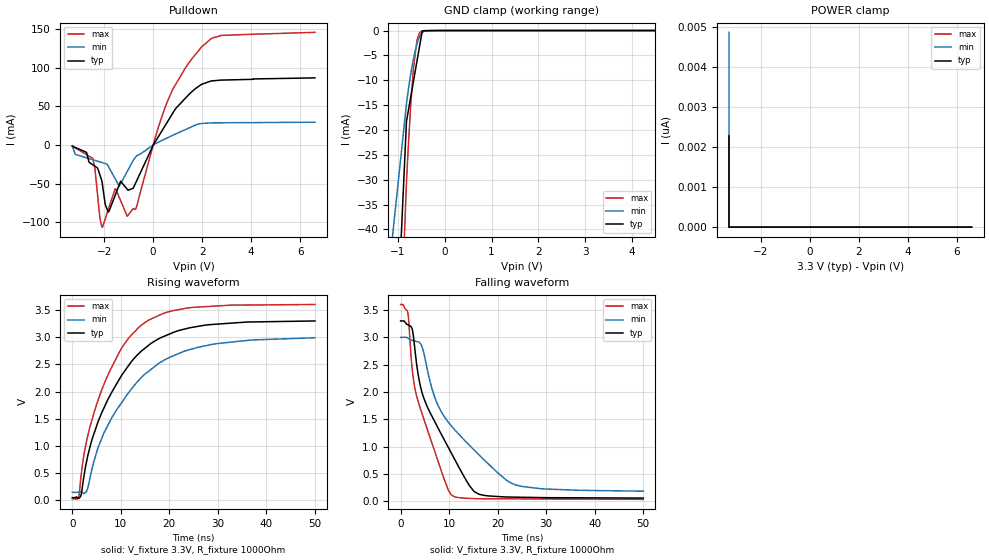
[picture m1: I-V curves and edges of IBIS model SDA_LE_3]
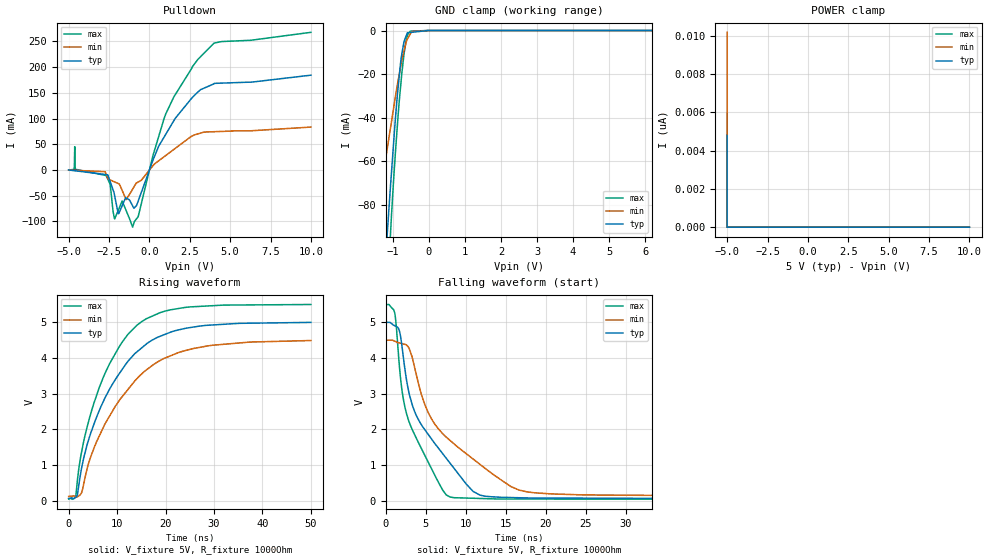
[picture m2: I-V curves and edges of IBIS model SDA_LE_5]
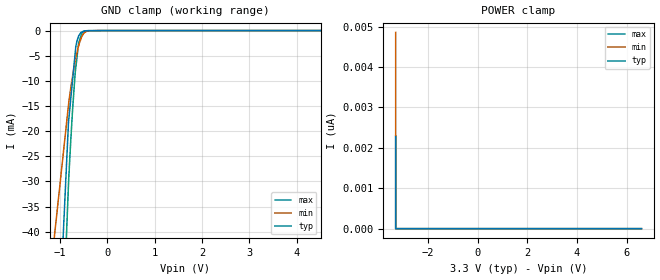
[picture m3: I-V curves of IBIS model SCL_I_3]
| Texas Instruments Incorporated
| Low-Power Bidirectional I2C Isolators
| Marketing part#   Voltage Range   Package-type   #pins/pkg drawing
| ISO1541D   3V-5.5V   SOIC   8-pin D
[IBIS Ver]   4.1
[File name]   iso1541.ibs
[File Rev]   1.0
[Date]   06/21/2012
[Source]   TIspiceD simulations
   Texas Instruments Incorporated.
   Analog eLab Design Center, HPA
   12500 TI Blvd
   Dallas, TX -75243
   For Support e-mail: elab_scm_ibis@list.ti.com
[Notes]   Revision History:
   Rev 1.0: 06/21/2012
   - C_comp although listed in numerical order of value are
   obtained from varying PVT conditions.
   For PVT conditions for each specific value, refer to the
   buffer description under respective [Model].
   IBIS model user is responsible for using appropriate
   C_comp to simulate for Signal Integrity.
   - IBIS model matched to TISPICED simulations
   - Pulldown data is non-monotonic, reflects circuit behavior
[Disclaimer] This model is designed as an aid for customers of Texas Instruments.
 TI and its licensors and suppliers make no warranties, either expressed
 or implied, with respect to this  model, including the warranties of
 merchantability or fitness for a particular purpose.
 The model is provided solely on an "as is" basis. The entire risk as to
 its quality and performance is with the customer.
[Copyright] (C)Copyright 2012 Texas Instruments Incorporated.
   All rights reserved.
|   Component ISO1541D
[Component]   ISO1541D
[Manufacturer]  Texas Instruments Incorporated
[Package]   |SOIC (D) 8-pin
|   typ   min   max
R_pkg   0.06626   0.03167   0.11324
L_pkg   2.49942nH   2.25405nH   2.79138nH
C_pkg   0.41610pF   0.38404pF   0.69535pF
[Pin]   signal_name   model_name   R_pin   L_pin   C_pin
1   VCC1   POWER   0.03718  2.27597n  0.43076p
2   SDA1   SDA_LE   0.09214  2.47816n  0.38404p
3   SCL1   SCL_I   0.11324  2.79138n  0.40143p
4   GND1   GND   0.03348  2.51166n  0.69535p
5   GND2   GND   0.03167  2.53947n  0.67094p
6   SCL2   SCL_O   0.09215  2.48718n  0.38609p
7   SDA2   SDA_RI   0.11323  2.77707n  0.39917p
8   VCC2   POWER   0.04038  2.25405n  0.46007p
[Model Selector] SDA_LE
SDA_LE_3   SDA I/O left side model for 3.0V - 3.6V
SDA_LE_5   SDA I/O left side model for 4.5V - 5.5V
[Model Selector] SDA_RI
SDA_RI_3   SDA I/O right side model for 3.0V - 3.6V
SDA_RI_5   SDA I/O right side model for 4.5V - 5.5V
[Model Selector] SCL_I
SCL_I_3   SDA Input left side model for 3.0V - 3.6V
SCL_I_5   SDA Input left side model for 4.5V - 5.5V
[Model Selector] SCL_O
SCL_O_3   SDA Output right side model for 3.0V - 3.6V
SCL_O_5   SDA Output right side model for 4.5V - 5.5V
| Models and submodels in the file (8): SDA_LE_3 (I/O_open_drain), SDA_LE_5 (I/O_open_drain), SCL_I_3 (Input), SCL_I_5 (Input), SDA_RI_3 (I/O_open_drain), SDA_RI_5 (I/O_open_drain), SCL_O_3 (Open_drain), SCL_O_5 (Open_drain)
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|   SDA Left 3.3V I/O Model
[Model]   SDA_LE_3
Model_type   I/O_open_drain
Polarity   Non-Inverting
Enable   Active-Low
Vinl = 0.5
Vinh = 2.52
Vmeas = 1.65
Vref = 1.65
Cref = 15pF
Rref = 1000
|   typ   min   max
|   (nom PVT)   (fast PVT)   (slow PVT)
C_comp   4.033p   3.367p   4.533p
|C_comp (High state)   4.033p   3.367p   4.533p
|C_comp (Low state)   5.596p   4.907p   5.983p
|PVT   Nom   Slow   Fast
[Voltage Range]   3.3   3   3.6
[Temperature Range]   27   136   -40
[Pullup Reference]   3.3   3   3.6
[Pulldown Reference]   -0   -0   -0
[Power Clamp Reference]   3.3   3   3.6
[GND Clamp Reference]   -0   -0   -0
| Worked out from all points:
|   slope of the pulldown table from 0 to 0.495 V, typ, clamps not added: 19.4 ohm
|   GND clamp passes 1 mA (typ) near -0.50 V on its own axis
|   falling waveform, V_fixture 3.3V, R_fixture 1000Ohm: 20-80 % time 8.4ns typ, 11.9ns min, 5.69ns max; typ from 3.3 V to 0.057 V
|   rising waveform, V_fixture 3.3V, R_fixture 1000Ohm: 20-80 % time 10.2ns typ, 12ns min, 8.59ns max; typ from 0.053 V to 3.3 V
[Pulldown]
|   Voltage   I(typ)   I(min)   I(max)
-3.3V     -1.441mA   -854.9uA   -1.481mA
-2.462V   -25.48mA   -19.01mA   -17.28mA
-2.095V   -46.15mA   -22.58mA   -105.6mA
-1.835V   -86.44mA   -27.36mA   -83.61mA
-1.533V   -63.51mA   -44.52mA   -56.4mA
-1.329V   -46.75mA   -49.98mA   -71.69mA
-1.058V   -57.16mA   -34.04mA   -92.04mA
-665.1mV  -45.59mA   -13.84mA   -78.65mA
800.2mV   41.16mA    12.55mA    72.1mA
1.984V    78.4mA     27.85mA    126.9mA
2.741V    83.72mA    28.65mA    141.4mA
6.6V      86.64mA    29.42mA    145.4mA
[GND Clamp]
|   Voltage   I(typ)   I(min)   I(max)
-3.3V     -815.4mA   -640mA     -971mA
-1.208V   -99.67mA   -49.74mA   -133.4mA
-1.091V   -75.48mA   -39.34mA   -97.6mA
-816.4mV  -18.3mA    -14.78mA   -30.7mA
-780mV    -16.34mA   -12.22mA   -23.92mA
-720.5mV  -13.12mA   -8.521mA   -14.39mA
-665.1mV  -10.12mA   -5.641mA   -7.366mA
-591.4mV  -6.144mA   -2.677mA   -1.944mA
-551.3mV  -3.973mA   -1.563mA   -734.8uA
-478.8mV  -55.54uA   -412.4uA   -98.93uA
-198.6mV  -17.66uA   -327nA     -154.7nA
6.6V      0A         0A         0A
[POWER Clamp]
|   Voltage   I(typ)   I(min)   I(max)
-3.3V     2.274nA    4.859nA    2.297nA
-3.3V     0A         0A         0A
-3.3V     0A         0A         0A
6.6V      0A         0A         0A
[Ramp]
R_load = 1000
|   typ   min   max
dV/dt_r   1.94673/1.02316e-08   1.70302/1.18334e-08   2.14001/8.58161e-09
dV/dt_f   1.9456/8.391e-09   1.69022/1.18691e-08   2.13948/5.67055e-09
[Falling Waveform]
V_fixture = 3.3V
V_fixture_min = 3V
V_fixture_max = 3.6V
R_fixture = 1000Ohm
C_fixture = 0F
|   Time   V(typ)   V(min)   V(max)
0s        3.3V       3V         3.6V
1.498ns   3.229V     2.986V     3.446V
2.486ns   3.108V     2.942V     2.34V
3.414ns   2.436V     2.921V     1.888V
5.316ns   1.765V     2.49V      1.361V
7.433ns   1.387V     1.809V     805.8mV
10.44ns   882.6mV    1.38V      115.5mV
15.14ns   177.9mV    938.5mV    48mV
23.88ns   73.47mV    293.4mV    42.9mV
50ns      57.34mV    183mV      34.2mV
[Rising Waveform]
V_fixture = 3.3V
V_fixture_min = 3V
V_fixture_max = 3.6V
R_fixture = 1000Ohm
C_fixture = 0F
|   Time   V(typ)   V(min)   V(max)
0s        52.63mV    150.1mV    32.79mV
1.366ns   41.87mV    157.1mV    77.54mV
1.856ns   113mV      153.4mV    486.1mV
2.88ns    687.9mV    157.4mV    1.06V
6.136ns   1.625V     1.156V     2.046V
9.812ns   2.245V     1.751V     2.744V
13.76ns   2.704V     2.214V     3.185V
18.88ns   3.014V     2.576V     3.44V
25.88ns   3.197V     2.813V     3.552V
50ns      3.297V     2.988V     3.599V
|   SDA Left 5V I/O Model
[Model]   SDA_LE_5
Model_type   I/O_open_drain
Polarity   Non-Inverting
Enable   Active-Low
Vinl = 0.5
Vinh = 3.85
Vmeas = 2.5
Vref = 2.5
Cref = 15pF
Rref = 1000
|   typ   min   max
|   (nom PVT)   (fast PVT)   (slow PVT)
C_comp   3.824p   3.201p   4.341p
|C_comp (ON state)   3.824p   3.201p   4.341p
|C_comp (OFF state)   4.090p   3.369p   4.747p
|PVT   Nom   Slow   Fast
[Voltage Range]   5   4.5   5.5
[Temperature Range]   27   136   -40
[Pullup Reference]   5   4.5   5.5
[Pulldown Reference]   -0   -0   -0
[Power Clamp Reference]   5   4.5   5.5
[GND Clamp Reference]   -0   -0   -0
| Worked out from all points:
|   slope of the pulldown table from 0 to 0.75 V, typ, clamps not added: 13.5 ohm
|   GND clamp passes 1 mA (typ) near -0.59 V on its own axis
|   falling waveform, V_fixture 5V, R_fixture 1000Ohm: 20-80 % time 5.86ns typ, 8.17ns min, 3.71ns max; typ from 5 V to 0.061 V
|   rising waveform, V_fixture 5V, R_fixture 1000Ohm: 20-80 % time 10ns typ, 11.6ns min, 8.51ns max; typ from 0.058 V to 5 V
[Pulldown]
|   Voltage   I(typ)   I(min)   I(max)
-5V       114.9uA    34.82uA    189.2uA
-4.66V    -1.19mA    -456.2uA   1.163mA
-4.624V   -1.328mA   -507.9uA   45.41mA
-4.584V   -1.482mA   -565.8uA   1.547mA
-2.677V   -8.802mA   -8.11mA    -10.73mA
-2.169V   -47.15mA   -22.82mA   -93.81mA
-1.93V    -84.92mA   -26.14mA   -78.43mA
-1.686V   -69.33mA   -39.6mA    -60.1mA
-1.039V   -69.58mA   -37.18mA   -111mA
1.024V    70.1mA     28.52mA    109.9mA
2.995V    151.3mA    70.22mA    214.8mA
10V       184.4mA    83.55mA    267.7mA
[GND Clamp]
|   Voltage   I(typ)   I(min)   I(max)
-5V       -1.078A    -841.4mA   -1.257A
-1.536V   -182.6mA   -122mA     -238.4mA
-1.234V   -111.6mA   -63.88mA   -147.4mA
-1.215V   -106.8mA   -60.09mA   -141mA
-1.108V   -80.87mA   -48.84mA   -105.3mA
-1.073V   -72.38mA   -45.15mA   -94.57mA
-911.4mV  -36.12mA   -28.15mA   -51.25mA
-767.8mV  -12.11mA   -14.79mA   -22.09mA
-695.2mV  -5.155mA   -9.331mA   -10.98mA
-638.6mV  -2.707mA   -5.775mA   -4.887mA
-516.2mV  -876.4uA   -1.491mA   -277.5uA
10V       0A         0A         0A
[POWER Clamp]
|   Voltage   I(typ)   I(min)   I(max)
-5V       4.793nA    10.19nA    5.967nA
-5V       0A         0A         0A
-5V       0A         0A         0A
10V       0A         0A         0A
[Ramp]
R_load = 1000
|   typ   min   max
dV/dt_r   2.96373/1.0022e-08   2.62546/1.15746e-08   3.27428/8.51231e-09
dV/dt_f   2.96329/5.82536e-09   2.62267/8.14594e-09   3.2739/3.70478e-09
[Falling Waveform]
V_fixture = 5V
V_fixture_min = 4.5V
V_fixture_max = 5.5V
R_fixture = 1000Ohm
C_fixture = 0F
|   Time   V(typ)   V(min)   V(max)
0s        5V         4.5V       5.5V
1.116ns   4.906V     4.473V     5.271V
1.99ns    4.392V     4.406V     3.159V
2.813ns   3.125V     4.308V     2.279V
3.802ns   2.399V     3.552V     1.764V
5.274ns   1.872V     2.489V     1.1V
8.039ns   1.056V     1.693V     109.3mV
11.79ns   160.4mV    1.021V     67.6mV
17.66ns   83.02mV    252.6mV    51.97mV
50ns      61.18mV    128.9mV    43.5mV
[Rising Waveform]
V_fixture = 5V
V_fixture_min = 4.5V
V_fixture_max = 5.5V
R_fixture = 1000Ohm
C_fixture = 0F
|   Time   V(typ)   V(min)   V(max)
0s        57.65mV    113mV      42.31mV
1.449ns   85.7mV     109.5mV    119.9mV
3.02ns    1.136V     406.6mV    1.605V
4.453ns   1.844V     1.19V      2.385V
6.324ns   2.525V     1.81V      3.171V
10.37ns   3.545V     2.791V     4.298V
13.98ns   4.158V     3.402V     4.904V
18.66ns   4.596V     3.913V     5.257V
25.66ns   4.864V     4.262V     5.436V
50ns      4.997V     4.489V     5.499V
|   SCL_I Left 3.3V Input Model
[Model]   SCL_I_3
Model_type   Input
Polarity   Non-Inverting
Enable   Active-Low
Vinl = 0.5
Vinh = 2.52
|   typ   min   max
|   (nom PVT)   (fast PVT)   (slow PVT)
C_comp   4.033p   3.367p   4.533p
|PVT   Nom   Slow   Fast
[Voltage Range]   3.3   3   3.6
[Temperature Range]   27   136   -40
[Power Clamp Reference]   3.3   3   3.6
[GND Clamp Reference]   -0   -0   -0
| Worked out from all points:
|   GND clamp passes 1 mA (typ) near -0.60 V on its own axis
[GND Clamp]
|   Voltage   I(typ)   I(min)   I(max)
-3.3V     -815.4mA   -640mA     -971mA
-1.192V   -94.35mA   -47.93mA   -128.9mA
-1.071V   -69.74mA   -37.22mA   -91.67mA
-816.3mV  -18.29mA   -14.83mA   -30.59mA
-729.1mV  -9.771mA   -9.045mA   -15.66mA
-675.3mV  -4.514mA   -6.13mA    -8.488mA
-660.7mV  -3.088mA   -5.437mA   -7.28mA
-602.7mV  -1.096mA   -3.08mA    -2.475mA
-550.1mV  -339uA     -1.535mA   -982.6uA
-439.1mV  -49.92uA   -175uA     -33.86uA
-236mV    -24.2uA    -1.134uA   -1.981uA
6.6V      0A         0A         0A
[POWER Clamp]
|   Voltage   I(typ)   I(min)   I(max)
-3.3V     2.274nA    4.859nA    2.297nA
-3.3V     0A         0A         0A
-3.3V     0A         0A         0A
6.6V      0A         0A         0A
